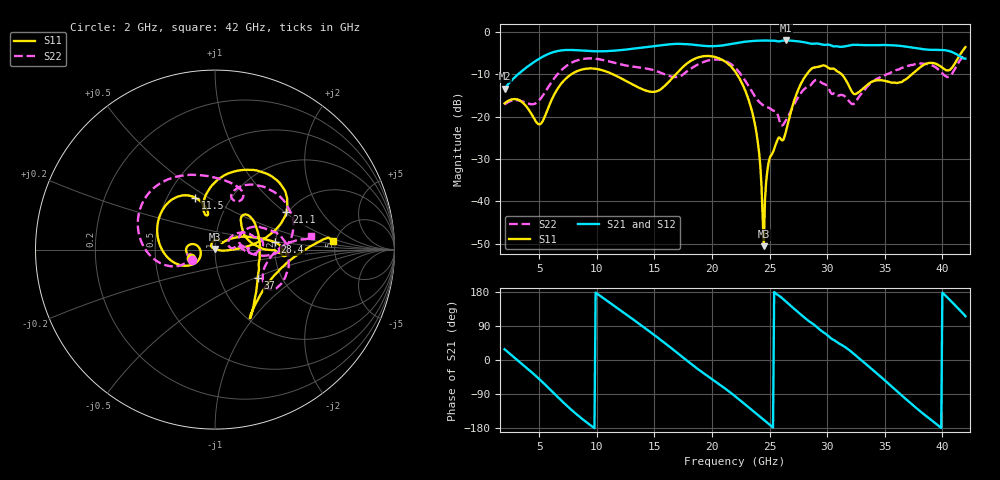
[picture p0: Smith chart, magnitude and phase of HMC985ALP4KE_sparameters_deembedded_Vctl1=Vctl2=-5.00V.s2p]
!s2p File: Measurements: S11, S21, S12, S22
# GHz S dB R 50.0
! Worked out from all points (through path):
!   401 points, 2 GHz to 42 GHz, reference 50 ohm
!   highest |S21| = -2.05 dB at 26.4 GHz (marker M1); lowest = -13.4 dB at 2 GHz (marker M2)
!   lowest |S11| = -50.6 dB at 24.5 GHz (marker M3), VSWR 1.01, Z = 49.9 + j0.283 ohm
!   |S11| at or under -10 dB: start of sweep to 7.811 GHz; 22.16 GHz to 28.24 GHz (6.077 GHz wide, 24.1 % of centre); 31.24 GHz to 37.37 GHz (6.134 GHz wide, 17.9 % of centre)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
!   |S22| runs from -22.1 to -5.3 dB; largest |S21 - S12| = 0.00091
!   S11 on the Smith chart (normalised r, x): 2 GHz: 0.76, -0.07; 11.5 GHz: 0.68, +0.44; 21.1 GHz: 1.97, +1.03; 28.4 GHz: 2.00, +0.18; 37 GHz: 1.52, -0.52; 42 GHz: 4.75, +0.80
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2  -16.88 -161.7  -13.43 28.3  -13.43 28.3  -17.18 -155.5
5  -21.84 -172.4  -6.37 -50.1  -6.37 -50.1  -16.18 -159.7
6.3  -14.85 -150.2  -4.75 -88.3  -4.76 -88.3  -11.02 -161.5
8.7  -8.91 150.4  -4.44 -154.5  -4.44 -154.5  -6.46 151.3
11.5  -10.16 111.1  -4.47 143.2  -4.47 143.2  -7.30 105.1
13.6  -13.11 101.1  -3.85 97.2  -3.85 97.2  -8.39 75.7
15.4  -13.82 105.8  -3.26 56.5  -3.26 56.6  -9.49 62.0
17.9  -7.34 80.3  -2.94 -3.4  -2.94 -3.4  -9.21 72.0
21.1  -6.95 27.7  -3.14 -74.3  -3.14 -74.2  -6.85 16.1
22  -9.33 17.1  -2.71 -95.4  -2.71 -95.4  -8.44 0.6
23.6  -20.16 -0.0  -2.17 -135.1  -2.17 -135.1  -14.70 -4.6
24.5  -50.56 106.8  -2.08 -157.8  -2.08 -157.7  -17.40 7.8
25  -29.86 132.9  -2.10 -170.5  -2.10 -170.5  -18.00 10.8
26.4  -23.80 41.5  -2.06 154.8  -2.05 154.8  -20.99 32.6
28.4  -9.43 7.0  -2.70 102.8  -2.70 102.9  -12.85 18.3
28.7  -8.60 2.1  -2.84 96.6  -2.85 96.6  -12.18 16.3
30.7  -8.95 -3.0  -3.44 50.7  -3.44 50.7  -14.52 2.1
32.5  -14.64 31.1  -3.09 11.1  -3.09 11.1  -16.45 27.3
35.4  -11.83 19.4  -3.15 -64.4  -3.15 -64.4  -9.80 19.4
37  -10.88 -33.5  -3.57 -107.5  -3.57 -107.5  -8.06 5.0
39.8  -8.07 -57.7  -4.29 -177.0  -4.28 -176.9  -9.24 -36.1
42  -3.60 4.1  -6.33 115.3  -6.33 115.3  -5.35 8.3
